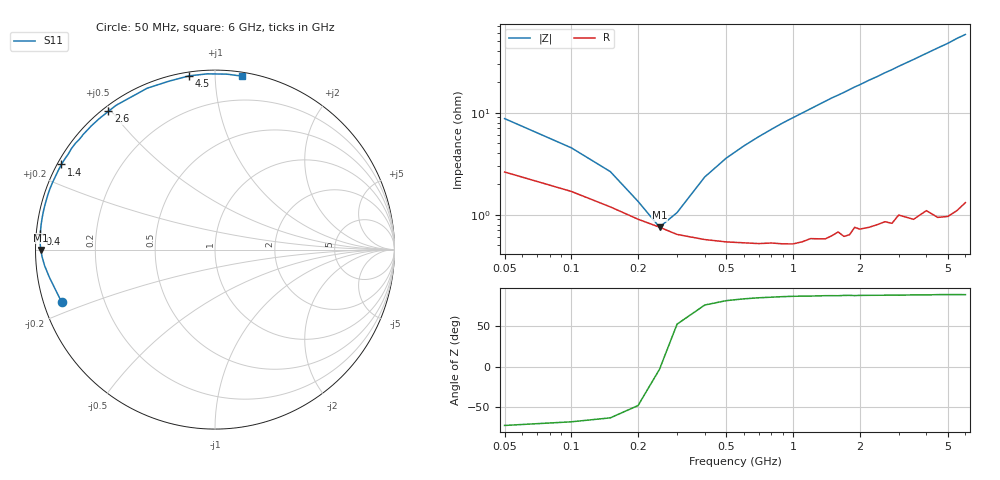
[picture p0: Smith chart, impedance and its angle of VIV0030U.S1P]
! Infineon Technologies  Discrete & RF Semiconductors
! BB 804
! Si Tuning Diode in SOT23
! VR =
! S-Parameters:  July  1999
# GHz  S  MA  R  50
!  f  S11
! GHz  MAG  ANG
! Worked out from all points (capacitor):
!   34 points, 50 MHz to 6 GHz, reference 50 ohm
!   read as one part to ground: C = 320 pF near 50 MHz
!   lowest |Z| = 754 mohm at 250 MHz (marker M1)
!   series resonance near 252.5 MHz, so ESL is about 1.2 nH
!   S11 on the Smith chart (normalised r, x): 50 MHz: 0.05, -0.17; 400 MHz: 0.01, +0.05; 1.4 GHz: 0.01, +0.26; 2.6 GHz: 0.02, +0.49; 4.5 GHz: 0.02, +0.86; 6 GHz: 0.03, +1.17
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0.05  0.903 -161.0
0.1  0.9351 -170.4
0.15  0.9536 -174.6
0.2  0.9646 -177.7
0.25  0.9703 -179.9
0.3  0.9748 178.1
0.4  0.9775 174.8
0.5  0.9787 171.9
0.6  0.9792 169.3
0.8  0.9795 164.4
0.9  0.98 162.0
1.1  0.9794 157.6
1.4  0.9786 151.0
1.6  0.9755 146.9
1.7  0.978 144.9
1.9  0.9737 140.7
2  0.975 138.9
2.2  0.9747 134.9
2.4  0.9739 131.4
2.6  0.9729 127.6
2.8  0.9746 124.3
3  0.9705 120.7
3.5  0.9754 112.8
4  0.9727 105.3
4.5  0.9787 98.5
5  0.9802 92.5
5.5  0.9798 86.1
6  0.9781 81.1
